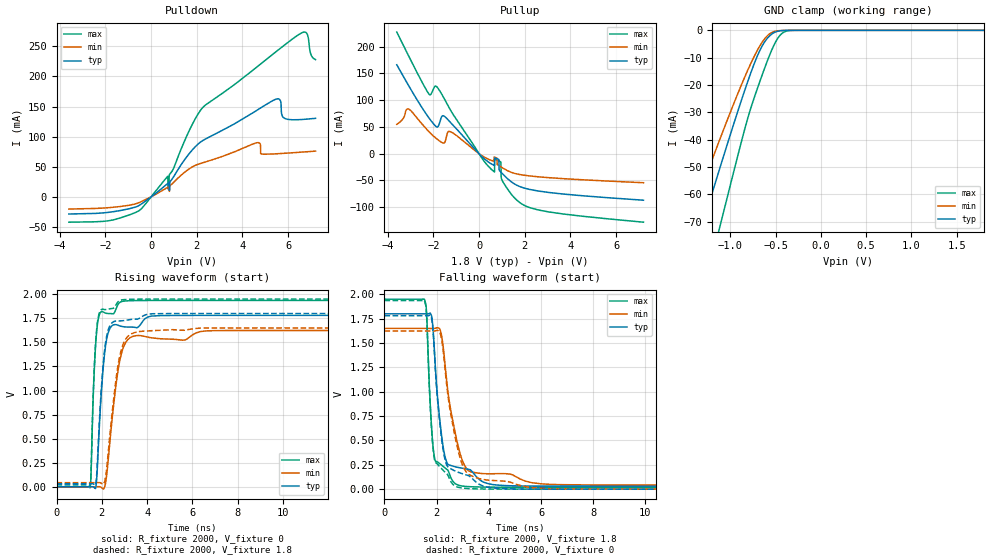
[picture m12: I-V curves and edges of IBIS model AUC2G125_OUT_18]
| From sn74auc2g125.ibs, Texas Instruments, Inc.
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[Model]   AUC2G125_OUT_18
Model_type  3-state
Enable   Active-Low
Vref =   0
Rref =   1000
Cref =   30p
Vmeas =   0.9
| variable   typ   min   max
C_comp   5.16pF   4.61pF   5.42pF
| C_pullup   5.87pF   1.37pF   12.96pF
| C_pulldown   6.42pF   5.22pF   15.40pF
| C_tri-state   5.16pF   4.61pF   5.42pF
[Temperature Range]   40   100   -40
| Ambient temperature   25   85   -40
[Voltage range]   1.8   1.65   1.95
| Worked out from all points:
|   slope of the pulldown table from 0 to 0.27 V, typ, clamps not added: 34.3 ohm
|   slope of the pullup table from 0 to 0.27 V, typ, clamps not added: 24.6 ohm
|   GND clamp passes 1 mA (typ) near -0.53 V on its own axis
|   rising waveform, R_fixture 2000, V_fixture 0: 20-80 % time 308ps typ, 484ps min, 195ps max; typ from 0 V to 1.78 V
|   falling waveform, R_fixture 2000, V_fixture 1.8: 20-80 % time 371ps typ, 597ps min, 225ps max; typ from 1.8 V to 0.031 V
|   rising waveform, R_fixture 2000, V_fixture 1.8: 20-80 % time 307ps typ, 480ps min, 194ps max; typ from 0.031 V to 1.8 V
|   falling waveform, R_fixture 2000, V_fixture 0: 20-80 % time 371ps typ, 594ps min, 225ps max; typ from 1.78 V to 0 V
[GND Clamp]
| AUC2G125_OUT_18
|   Voltage   I(typ)   I(min)   I(max)
-3.6V     -324.8mA   -272.6mA   -395.3mA
-1.48V    -89.78mA   -72.17mA   -119.8mA
-1.435V   -84.84mA   -68.08mA   -113.9mA
-1.3V     -70.1mA    -55.95mA   -96.04mA
-1.105V   -49.1mA    -38.82mA   -70.28mA
-830mV    -20.77mA   -16.17mA   -34.67mA
-685mV    -8.07mA    -6.262mA   -19.65mA
-565mV    -1.967mA   -1.239mA   -8.908mA
-490mV    -465.2uA   -242.6uA   -3.617mA
-425mV    -91.43uA   -52.01uA   -990.1uA
-300mV    -2.28uA    -2.125uA   -16.99uA
1.8V      471.3pA    37.82nA    526.5pA
[Pulldown]
| AUC2G125_OUT_18
|   Voltage   I(typ)   I(min)   I(max)
-3.6V     -28.49mA   -20.22mA   -42.08mA
-710mV    -17.24mA   -11.96mA   -26.36mA
730mV     22.14mA    15.83mA    34.29mA
780mV     23.67mA    17.08mA    13.96mA
805mV     10.91mA    9.302mA    37.17mA
2.23V     92.83mA    56.26mA    147.2mA
4.65V     144.3mA    90.06mA    216.4mA
5.505V    162.8mA    71.64mA    242.3mA
5.79V     131.9mA    72.29mA    250.8mA
6.445V    128.2mA    73.96mA    269.3mA
6.815V    129.2mA    74.96mA    271.7mA
7.2V      130.5mA    76.01mA    228mA
[Pullup]
| AUC2G125_OUT_18
|   Voltage   I(typ)   I(min)   I(max)
-3.6V     166.1mA    54.83mA    227.3mA
-3.08V    127.2mA    83.38mA    182.7mA
-2.18V    66.16mA    40.7mA     110.8mA
-1.91V    51.96mA    29.83mA    126.4mA
-1.51V    69.63mA    20.5mA     101.9mA
-1.25V    58.38mA    41.07mA    81.58mA
385mV     -14.76mA   -9.808mA   -22.53mA
870mV     -11.11mA   -22.27mA   -13.48mA
955mV     -34.36mA   -24.54mA   -15.75mA
1.015V    -36.99mA   -26.15mA   -50.39mA
1.755V    -60.96mA   -38.77mA   -90.45mA
7.2V      -86.99mA   -54.32mA   -128.1mA
[Ramp]
| AUC2G125_OUT_18
| variable   typ   min   max
dV/dt_r   1.08/3.11E-10   0.99/4.92E-10   1.17/1.96E-10
dV/dt_f   1.07/3.71E-10   0.97/6.03E-10   1.16/2.30E-10
R_load = 2000
[Rising Waveform]
| AUC2G125_OUT_18
R_fixture =   2000
C_fixture =   0
L_fixture =   0
V_fixture =   0
V_fixture_min = 0
V_fixture_max = 0
|   Time   V(typ)   V(min)   V(max)
0s        8.423nV    29.16nV    1.166nV
1.48ns    131uV      -8.259uV   -11.51mV
1.645ns   -4.146mV   18.84uV    1.086V
1.755ns   28.65mV    399.6uV    1.565V
2.105ns   1.343V     -15.54mV   1.811V
2.36ns    1.646V     472.7mV    1.799V
2.86ns    1.667V     1.377V     1.923V
3.41ns    1.658V     1.565V     1.934V
6.615ns   1.78V      1.619V     1.936V
20ns      1.78V      1.624V     1.936V
[Falling Waveform]
| AUC2G125_OUT_18
R_fixture =   2000
C_fixture =   0
L_fixture =   0
V_fixture =   1.8
V_fixture_min = 1.65
V_fixture_max = 1.95
|   Time   V(typ)   V(min)   V(max)
0s        1.8V       1.65V      1.95V
1.535ns   1.8V       1.65V      1.946V
1.61ns    1.8V       1.65V      1.822V
1.81ns    1.773V     1.649V     618.1mV
1.92ns    1.403V     1.65V      321.7mV
2.29ns    372.3mV    1.368V     224.4mV
2.815ns   223.5mV    452.6mV    42.64mV
3.26ns    201.2mV    182.8mV    25.82mV
5.97ns    31.64mV    55.6mV     19.59mV
20ns      30.97mV    42.25mV    19.49mV
[Rising Waveform]
| AUC2G125_OUT_18
R_fixture =   2000
C_fixture =   0
L_fixture =   0
V_fixture =   1.8
V_fixture_min = 1.65
V_fixture_max = 1.95
|   Time   V(typ)   V(min)   V(max)
0s        30.94mV    42.24mV    19.47mV
1.48ns    31.07mV    42.23mV    8.597mV
1.52ns    31.21mV    42.23mV    124.3mV
1.62ns    30.43mV    42.23mV    954.2mV
1.725ns   17.52mV    42.44mV    1.489V
1.875ns   592.8mV    42.97mV    1.793V
2.17ns    1.502V     107.6mV    1.841V
2.81ns    1.723V     1.375V     1.936V
3.825ns   1.775V     1.616V     1.949V
20ns      1.8V       1.65V      1.95V
[Falling Waveform]
| AUC2G125_OUT_18
R_fixture =   2000
C_fixture =   0
L_fixture =   0
V_fixture =   0
V_fixture_min = 0
V_fixture_max = 0
|   Time   V(typ)   V(min)   V(max)
0s        1.78V      1.624V     1.936V
1.535ns   1.78V      1.624V     1.931V
1.61ns    1.78V      1.624V     1.806V
1.81ns    1.751V     1.623V     599.3mV
1.915ns   1.398V     1.623V     310.3mV
2.28ns    355.7mV    1.351V     184.8mV
2.79ns    177.2mV    434.7mV    22.28mV
3.24ns    135.9mV    149.5mV    6.16mV
5.715ns   856.7uV    14.42mV    127.5uV
20ns      32.2uV     9.742uV    13.53uV
